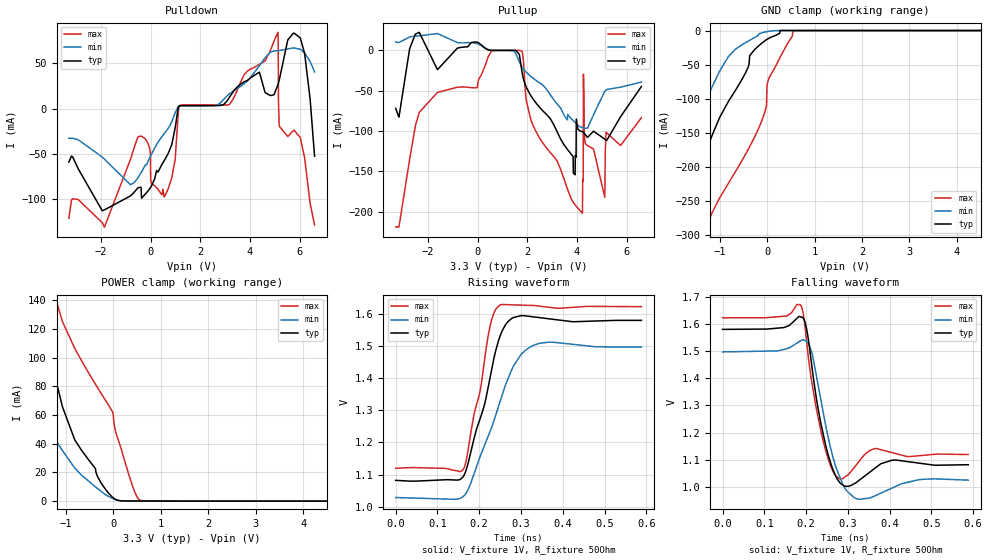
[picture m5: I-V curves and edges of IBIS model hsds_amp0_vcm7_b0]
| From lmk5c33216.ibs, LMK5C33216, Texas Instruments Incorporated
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[Model]   hsds_amp0_vcm7_b0
Model_type   Output
Polarity   Non-Inverting
Vmeas = 1.3
Vref = 1
Cref = 0pF
Rref = 50
|   typ   min   max
C_comp   0.65pF   0.575pF   0.725pF
[Voltage Range]   3.3   3.135   3.465
[Temperature Range]   50   135   -40
[Pullup Reference]   3.3   3.135   3.465
[Pulldown Reference]   0   0   -0
[Power Clamp Reference]   3.3   3.135   3.465
[GND Clamp Reference]   0   0   0
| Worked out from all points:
|   slope of the pulldown table from 0 to 0.495 V, typ, clamps not added: 18.3 ohm
|   slope of the pullup table from 0 to 0.495 V, typ, clamps not added: 50.9 ohm
|   falling waveform, V_fixture 1V, R_fixture 50Ohm: 20-80 % time 32ps typ, 37.3ps min, 31.3ps max; typ from 1.58 V to 1.08 V
|   rising waveform, V_fixture 1V, R_fixture 50Ohm: 20-80 % time 56.5ps typ, 77.5ps min, 41.4ps max; typ from 1.08 V to 1.58 V
[Pulldown]
|   Voltage   I(typ)   I(min)   I(max)
-3.3V     -59.03mA   -32.86mA   -121.2mA
-1.865V   -111.8mA   -55.91mA   -130.8mA
-815.1mV  -96.37mA   -84.03mA   -55.91mA
-221.1mV  -94.34mA   -62.53mA   -33.48mA
541.2mV   -57.54mA   -27.64mA   -97.49mA
1.155V    2.958mA    2.761mA    3.185mA
3.165V    12.05mA    16.12mA    4.541mA
5.125V    26.39mA    63.91mA    84.14mA
5.145V    28.25mA    63.97mA    9.214mA
5.184V    32.39mA    64.1mA     -19.66mA
6.026V    77.99mA    65.38mA    -32.08mA
6.6V      -52.62mA   40.53mA    -128.5mA
[GND Clamp]
|   Voltage   I(typ)   I(min)   I(max)
-3.3V     -892.9mA   -765.6mA   -1.068A
-1.924V   -314.6mA   -288.5mA   -459.9mA
-1.815V   -287mA     -251.4mA   -425.6mA
-1.478V   -218.2mA   -143.5mA   -333.1mA
-1.162V   -154.3mA   -82.94mA   -268mA
-815.1mV  -104mA     -38.12mA   -224.4mA
-171.6mV  -22.09mA   -4.573mA   -142.5mA
-13.2mV   -13.46mA   -1.685mA   -109.6mA
-3.3mV    -13.01mA   -1.546mA   -81.32mA
26.4mV    -11.77mA   -1.169mA   -72.35mA
551.1mV   0A         -83.65nA   -744.3uA
6.6V      0A         0A         0A
[Pullup]
|   Voltage   I(typ)   I(min)   I(max)
-3.3V     -71.9mA    10.56mA    -218.9mA
-2.35V    22.39mA    18.04mA    -76.91mA
570.9mV   -15.95uA   134.7uA    -438.5uA
1.789V    -26.34mA   -20.62mA   -1.283mA
3.858V    -152.4mA   -87.32mA   -188.6mA
4.224V    -100.8mA   -95.87mA   -201.9mA
4.254V    -101.3mA   -96.09mA   -162mA
4.264V    -101.5mA   -96.15mA   -29.54mA
4.333V    -104.3mA   -96.52mA   -114.6mA
5.125V    -110.1mA   -50.51mA   -182.3mA
5.174V    -111.5mA   -49.31mA   -101.9mA
6.6V      -44.75mA   -39.37mA   -83.41mA
[POWER Clamp]
|   Voltage   I(typ)   I(min)   I(max)
-3.3V     330.7mA    180mA      566.4mA
-2.736V   200mA      135.8mA    401.6mA
-1.647V   138.3mA    65.17mA    197.7mA
-1.459V   117.6mA    55.06mA    168.7mA
-1.082V   66.76mA    35.64mA    126mA
-815.1mV  42.67mA    23.06mA    106.5mA
-3.3mV    2.23mA     1.644mA    59.85mA
46.2mV    1.16mA     1.045mA    48.48mA
313.5mV   86.42uA    94.45uA    19.62mA
491.7mV   74.41uA    72.76uA    3.271mA
570.9mV   69.96uA    68.47uA    464.4uA
6.6V      0A         0A         0A
[Ramp]
R_load = 50
|   typ   min   max
dV/dt_r   0.29857/5.65288e-11   0.280859/7.7098e-11   0.301598/4.13634e-11
dV/dt_f   0.29857/3.17058e-11   0.282809/3.6024e-11   0.301598/3.11914e-11
[Falling Waveform]
V_fixture = 1V
V_fixture_min = 0.95V
V_fixture_max = 1.05V
R_fixture = 50Ohm
C_fixture = 0F
|   Time   V(typ)   V(min)   V(max)
0s        1.58V      1.497V     1.622V
186.2ps   1.626V     1.537V     1.671V
197.7ps   1.605V     1.539V     1.587V
209.3ps   1.499V     1.516V     1.432V
236ps     1.23V      1.316V     1.202V
257.4ps   1.096V     1.152V     1.083V
278.5ps   1.021V     1.046V     1.031V
327.2ps   1.025V     954.9mV    1.095V
405.4ps   1.099V     996.1mV    1.127V
588.4ps   1.082V     1.026V     1.12V
[Rising Waveform]
V_fixture = 1V
V_fixture_min = 0.95V
V_fixture_max = 1.05V
R_fixture = 50Ohm
C_fixture = 0F
|   Time   V(typ)   V(min)   V(max)
0s        1.082V     1.029V     1.12V
161.3ps   1.093V     1.032V     1.115V
168.6ps   1.114V     1.042V     1.142V
186.2ps   1.205V     1.097V     1.277V
202.2ps   1.275V     1.156V     1.361V
225.3ps   1.397V     1.232V     1.558V
247.3ps   1.521V     1.316V     1.625V
282.4ps   1.589V     1.438V     1.628V
334.9ps   1.59V      1.505V     1.626V
588.4ps   1.58V      1.497V     1.622V
